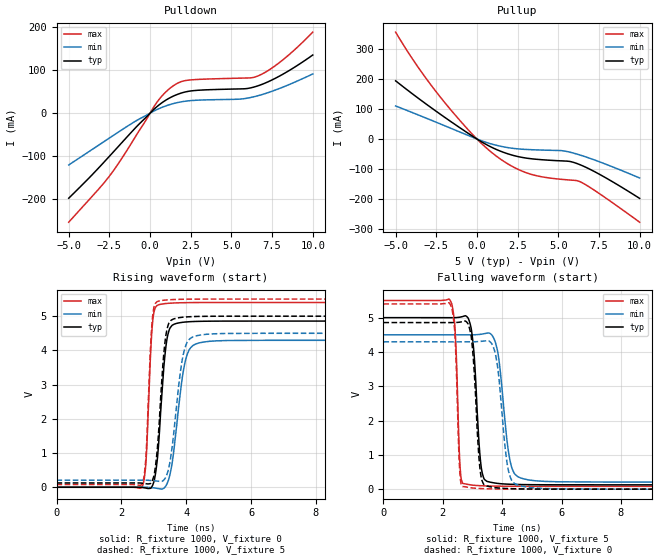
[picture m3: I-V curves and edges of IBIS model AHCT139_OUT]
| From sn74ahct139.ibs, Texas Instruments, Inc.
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[Model]   AHCT139_OUT
Model_type  Output
Vref =   0
Rref =   1000
Cref =   50p
Vmeas =   2.5
| variable   typ   min   max
C_comp   2.30pF   1.71pF   3.16pF
| C_pullup   2.50pF   1.76pF   3.16pF
| C_pulldown   2.10pF   1.71pF   2.47pF
[Temperature Range]   40   100   -40
| Ambient temperature   25   85   -40
[Voltage range]   5   4.5   5.5
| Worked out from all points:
|   slope of the pulldown table from 0 to 0.75 V, typ, clamps not added: 30.3 ohm
|   slope of the pullup table from 0 to 0.75 V, typ, clamps not added: 32.1 ohm
|   rising waveform, R_fixture 1000, V_fixture 0: 20-80 % time 223ps typ, 330ps min, 146ps max; typ from 0 V to 4.86 V
|   falling waveform, R_fixture 1000, V_fixture 5: 20-80 % time 197ps typ, 308ps min, 125ps max; typ from 5 V to 0.126 V
|   rising waveform, R_fixture 1000, V_fixture 5: 20-80 % time 215ps typ, 313ps min, 144ps max; typ from 0.126 V to 5 V
|   falling waveform, R_fixture 1000, V_fixture 0: 20-80 % time 193ps typ, 283ps min, 121ps max; typ from 4.86 V to 0 V
[Pulldown]
| AHCT139_OUT
|   Voltage   I(typ)   I(min)   I(max)
-5V       -197.5mA   -120.3mA   -253.2mA
-2.475V   -99.11mA   -57.09mA   -145mA
-1.545V   -60.56mA   -34.03mA   -93.77mA
355mV     12.95mA    7.146mA    21.7mA
795mV     25.94mA    14.45mA    42.62mA
1.265V    36.59mA    20.52mA    59.08mA
1.79V     45.13mA    25.4mA     71.35mA
2.3V      50.36mA    28.4mA     76.44mA
5.54V     56.36mA    32.68mA    81.35mA
6.6V      63.14mA    40.18mA    86.05mA
8.09V     88.91mA    59.36mA    121.6mA
10V       135.1mA    91.05mA    188.3mA
[Pullup]
| AHCT139_OUT
|   Voltage   I(typ)   I(min)   I(max)
-5V       193.5mA    109.9mA    355.5mA
-3.63V    136.5mA    80.49mA    239.8mA
-2.105V   76.82mA    46.85mA    129.6mA
-295mV    10.32mA    6.452mA    16.48mA
1.07V     -31.73mA   -19.13mA   -51.77mA
2.14V     -53.16mA   -30.5mA    -90.2mA
3.215V    -64.83mA   -35.2mA    -115.4mA
5.205V    -72.71mA   -38.73mA   -134.1mA
6.06V     -79.83mA   -48.75mA   -137.8mA
6.42V     -87.36mA   -54.67mA   -144.1mA
7.085V    -104.4mA   -66.92mA   -165.6mA
10V       -197.4mA   -129.5mA   -276.5mA
[Ramp]
| AHCT139_OUT
| variable   typ   min   max
dV/dt_r   2.93/2.31E-10   2.61/3.43E-10   3.26/1.52E-10
dV/dt_f   2.96/2.07E-10   2.61/3.23E-10   3.28/1.30E-10
R_load = 1000
[Rising Waveform]
| AHCT139_OUT
R_fixture =   1000
C_fixture =   0
L_fixture =   0
V_fixture =   0
V_fixture_min = 0
V_fixture_max = 0
|   Time   V(typ)   V(min)   V(max)
0s        1.341nV    2.225nV    826.5pV
2.63ns    -5.157mV   1.554mV    -4.567mV
2.755ns   -23.7mV    1.557mV    670.7mV
2.985ns   108mV      -15.79mV   4.999V
3.115ns   870.5mV    -34.39mV   5.319V
3.35ns    3.91V      7.088mV    5.367V
3.555ns   4.722V     638.1mV    5.382V
4.01ns    4.832V     3.821V     5.395V
4.7ns     4.853V     4.264V     5.399V
50ns      4.857V     4.295V     5.4V
[Falling Waveform]
| AHCT139_OUT
R_fixture =   1000
C_fixture =   0
L_fixture =   0
V_fixture =   5
V_fixture_min = 4.5
V_fixture_max = 5.5
|   Time   V(typ)   V(min)   V(max)
0s        5V         4.5V       5.5V
2.27ns    4.999V     4.5V       5.469V
2.415ns   5.001V     4.5V       4.635V
2.61ns    5.02V      4.5V       366.3mV
2.975ns   4.581V     4.5V       121mV
3.31ns    551.7mV    4.519V     99.24mV
3.87ns    166.1mV    3.901V     87.25mV
4.31ns    141.9mV    664.3mV    84.16mV
5.12ns    129.8mV    244.4mV    82.24mV
50ns      126.2mV    206.2mV    81.52mV
[Rising Waveform]
| AHCT139_OUT
R_fixture =   1000
C_fixture =   0
L_fixture =   0
V_fixture =   5
V_fixture_min = 4.5
V_fixture_max = 5.5
|   Time   V(typ)   V(min)   V(max)
0s        126.2mV    206.2mV    81.52mV
2.63ns    120.7mV    207.3mV    83.35mV
2.755ns   104.8mV    207mV      830.4mV
2.97ns    230.8mV    192.9mV    5.045V
3.11ns    1.129V     179.6mV    5.427V
3.305ns   3.856V     208.6mV    5.465V
3.47ns    4.802V     591.8mV    5.479V
3.95ns    4.974V     4.032V     5.495V
4.605ns   4.996V     4.469V     5.499V
50ns      5V         4.5V       5.5V
[Falling Waveform]
| AHCT139_OUT
R_fixture =   1000
C_fixture =   0
L_fixture =   0
V_fixture =   0
V_fixture_min = 0
V_fixture_max = 0
|   Time   V(typ)   V(min)   V(max)
0s        4.857V     4.295V     5.4V
2.26ns    4.856V     4.295V     5.372V
2.405ns   4.858V     4.295V     4.575V
2.595ns   4.873V     4.295V     281.9mV
2.955ns   4.473V     4.295V     38.79mV
3.285ns   388.2mV    4.309V     17.77mV
3.815ns   40.3mV     3.742V     6.197mV
4.235ns   16.56mV    454.6mV    2.982mV
5.02ns    4.154mV    39.75mV    867.2uV
50ns      1.117nV    1.045nV    864.8pV
